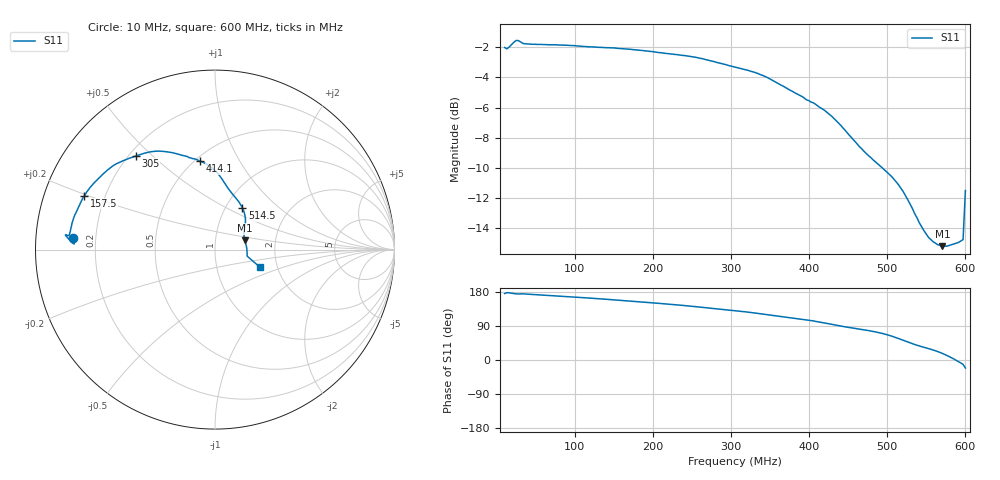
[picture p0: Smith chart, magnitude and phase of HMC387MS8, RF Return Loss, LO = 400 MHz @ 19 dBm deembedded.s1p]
!Hittite Microwave Corporation
!12 Elizabeth Drive
!Chelmsford, MA 01824
!Tel: 978-250-3343
!Fax: 978-250-3373
!Device: HMC387MS8, 450-500 MHz, GaAs MMIC High IP3 Mixer in 8-lead plastic SMT package
!Misc: RF Return Loss, LO = 400 MHz @ 19 dBm, Room
# MHZ S MA R 50
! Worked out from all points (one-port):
!   201 points, 10 MHz to 600 MHz, reference 50 ohm
!   lowest |S11| = -15.2 dB at 570.5 MHz (marker M1), VSWR 1.42, Z = 69.4 + j7.45 ohm
!   |S11| at or under -10 dB: 493.7 MHz to end of sweep
!   S11 on the Smith chart (normalised r, x): 10 MHz: 0.12, +0.04; 157.5 MHz: 0.12, +0.20; 305 MHz: 0.23, +0.44; 414.1 MHz: 0.53, +0.69; 514.5 MHz: 1.20, +0.60; 600 MHz: 1.62, -0.33
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10  0.793 175.4
12.95  0.785 177.7
15.9  0.796 177.3
24.75  0.837 174.5
27.7  0.836 174.3
33.6  0.818 174.5
45.4  0.813 173.3
83.75  0.808 168.2
157.5  0.787 157.5
192.9  0.772 151.9
231.25  0.751 145.4
263.7  0.728 138.9
305  0.683 130.2
340.4  0.641 121.2
378.75  0.567 110.7
414.15  0.501 99.8
428.9  0.469 94.1
452.5  0.403 85.3
470.2  0.359 79.6
496.75  0.311 68.4
514.45  0.278 56.6
526.25  0.248 47.4
541  0.208 37.0
552.8  0.186 30.1
570.5  0.174 17.4
582.3  0.176 5.8
597.05  0.183 -11.5
600  0.266 -21.1
